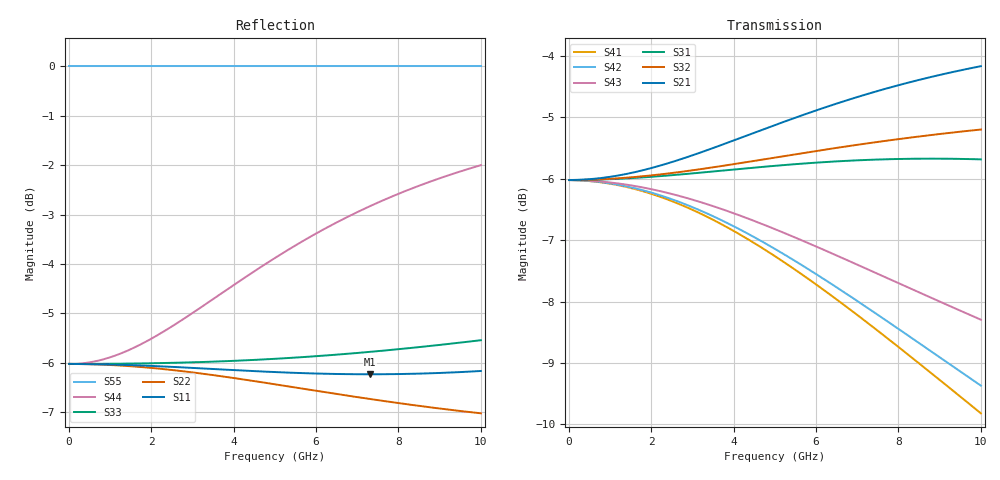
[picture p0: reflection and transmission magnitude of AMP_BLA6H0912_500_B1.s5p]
! Created Tue Apr 27 00:57:34 2010
# hz S ma R 50
! 5 Port Network Data from SP1.SP block
! freq  magS11  angS11  magS12  angS12  magS13  angS13  magS14  angS14
!  magS15  angS15
!  magS21  angS21  magS22  angS22  magS23  angS23
!  magS24  angS24  magS25  angS25
!  magS31  angS31  magS32  angS32
!  magS33  angS33  magS34  angS34  magS35  angS35
!  magS41  angS41
!  magS42  angS42  magS43  angS43  magS44  angS44  magS45  angS45
!  magS51  angS51  magS52  angS52  magS53  angS53  magS54  angS54
!  magS55  angS55
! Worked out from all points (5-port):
!   1000 points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, 10 MHz to 10 GHz, reference 50 ohm
!   strongest paths, dB at 10 MHz, 2.51 GHz, 5.01 GHz, 7.51 GHz, 10 GHz:
!     S21: -6.0, -5.7, -5.1, -4.6, -4.2
!     S32: -6.0, -5.9, -5.7, -5.4, -5.2
!     S31: -6.0, -5.9, -5.8, -5.7, -5.7
!     S43: -6.0, -6.2, -6.8, -7.6, -8.3
!     S42: -6.0, -6.3, -7.1, -8.2, -9.4
!     S41: -6.0, -6.4, -7.3, -8.5, -9.8
!   lowest |S11| = -6.2 dB at 7.31 GHz (marker M1), VSWR 2.91, Z = 20.1 + j19.2 ohm
!   |S11| at or under -10 dB: nowhere
